| IBIS File main_fixed.ibs
| Cadence Design Systems, Inc. 2024
|[Doc Num]   FPGA-MD-02062 1.2
[IBIS ver]   3.2
[File name]   machxo3d.ibs
[File Rev]   0.8
[Date]   Mon Sep 23 20:28:33 PDT 2024
[Source]   Lattice Semiconductor cs200fl Process
[Notes]   Device: LCMXO3D-4300HC   Final
   Device: LCMXO3D-4300ZC   Final
   Device: LCMXO3D-9400HC   Final
   Device: LCMXO3D-9400ZC   Final
   Device: LCMXO3D-9400HE   Final
   Device: LAMXO3D-4300HC   Final
   Device: LAMXO3D-4300ZC   Final
   Device: LAMXO3D-9400HC   Final
   Device: LAMXO3D-9400ZC   Final
   Device: LAMXO3D-9400HE   Final
   "Test Release - internal Lattice use ONLY"
   Lattice Semiconductor has worked hard to ensure the
   models below are accurate and complete.  However, the
   data below was generated using simulation of the
   input/output model files for the silicon.  Therefore,
   the data below is for reference and initial design
   purposes only.
   Lattice Semiconductor grants permission to use this
   data for use in printed circuit design using this
   Lattice programmable logic device.  Other use of this
   code, including the selling or duplication of any
   portion is strictly prohibited.
|   NAMING CONVENTION
   The IBIS [Model] header is limited by the specification to a
   total of characters.  With such a set of characters available
   for naming models it becomes important to attempt to
   meaningfully encode the IO standards so they fit within the
   twenty character limit.  It would seem that twenty characters
   would provide room enough for describing IO's.  However, the
   PLD IO structure continues to grow more and more complex.  The
   complexity is making the twenty characters insuffiently
   descriptive.  In order to overcome this issue the naming
   convention described below is implemented to resolve the issue.
The twenty character space is managed as follows:
   bbbvvvsdddprugtcoixx
   b = standard
   v = voltage (x.xx V)
   s = slew code
   d = drive (xx.x ma)
   p = pullup code
   r = series resistance  or bank_vccio code
   u = terminate to vcc code
   g = terminate to gnd code
   t = terminate to vtt code
   c = common mode termination mode
   o = diff resistor code
   i = diff resistor current code
   x = reserved
   standard
   LVCMOS   lvc
   lvcmosd   lvd
   lvcmosr   lvr
   LVDS25E   lve
   LVTTL   lvt
   lvttld   ltd
   PCI   pci
   pcix   pcx
   lvds25   lvs
   blvds25   blv
   blvds25e   blv
   mlvds25   mlv
   mlvds25e   mle
   lvpecl   lvp
   lvpecl33   lvp
   lvpecl33e   lvp
   cml   cml
   hypt   hyp
   rsds25   rsd
   rsds25e   rse
   mipi_lp   mip
   mipi   mip
   vref1   vr1
   vref2   vr2
   ref_res   rer
   i3c33   i3c
   i3c18   i3c
   i3c12   i3c
   slew
   na   a
   fast   f
   slow   s
   pullmode
   off   a
   pullup   b
   pulldown   c
   bushold   d
   clamp   e
   up_clamp   f
   down_clamp   g
   keeper_clamp   h
   i3c_clamp   e
   impedance or Bank_vccio
   off   a
   25   b
   33   c
   50   d
   100   e
   3.3   f
   2.5   g
   1.8   h
   1.5   i
   1.2   j
   termVCC
   off   a
   50   b
   100   c
   120   d
   termGND
   off   a
   50   b
   100   c
   120   d
   termVTT
   off   a
   60   b
   75   c
   120   d
   150   e
   210   f
   VCMT
   off   a
   VCMT   b
   VTT   c
   DDR-2   d
   differential resistor
   off   a
   100   b
   diff drive
   NA   a
   2.0   b
   3.5   c
   1.25   f
   2.5   g
   Reserved   IO type
   in   input only
   ou   output
   io   I/O
   od   Open drain
   ic   Inverting differential input
   (signal name only)
   it   Non-Inverting differential
   input (signal name only)
   on   Inverting differential output
   (signal name only)
   op   Non-Inverting differential output
   (signal name only)
   bn   Inverting differential I/O
   (signal name only)
   bp   Non-Inverting differential I/O
   (signal name only)
   Lattice Semiconductor Corporation
   5555 NE Moore Court
   Hillsboro, OR 97214
   U.S.A
   TEL: 1-800-Lattice (USA and Canada)
   408-826-6000 (other locations)
   web: http://www.latticesemi.com/
   email: techsupport@latticesemi.com
[Disclaimer]  This IBIS source code is intended as a design reference which
  illustrates how the Lattice Semiconductor device operates. It is the user's
  responsibility to verify their design for consistency and functionality
  through the use of formal verification methods. Lattice Semiconductor
  provides no warranty regarding the use or functionality of this data.
[Copyright] Copyright 2024 by Lattice Semiconductor Corporation
|   Component XO3D
[Component] XO3D
[Manufacturer] Lattice Semiconductor Corp.
[Package]
|CABGA484
|variable   typ   min   max
R_pkg   262.26m   144.47m   388.32m
L_pkg   4.725nH   1.887nH   8.095nH
C_pkg   0.7093pF   0.3624pF   1.17pF
|CABGA400
|varibale   typ   min   max
|R_pkg   249.7m   145.37m   389.76m
|L_pkg   4.325nH   1.917nH   7.316nH
|C_pkg   0.6713pF   0.3727pF   1.207pF
|CABGA256_9400
|varibale   typ   min   max
|R_pkg   230.24m   185.88m   297.14m
|L_pkg   3.46nH   2.215nH   5.403nH
|C_pkg   0.5928pF   0.3835pF   0.8599pF
|QFN72_9400
|varibale   typ   min   max
|R_pkg   149.35m   99.917m   233.44m
|L_pkg   2.376nH   1.45nH   3.785nH
|C_pkg   0.3325pF   0.2601pF   0.4543pF
|CABGA256_4300
|variable   typ   min   max
|R_pkg   275.2m   212.49m   370.68m
|L_pkg   4.143nH   2.728nH   6.386nH
|C_pkg   0.654pF   0.4691pF   0.909pF
|QFN72_4300
|variable   typ   min   max
|R_pkg   175.42m   121.83m   245.44m
|L_pkg   2.78nH   1.676nH   3.852nH
|C_pkg   0.3626pF   0.28pF   0.4651pF
|WLCSP69_9400
|variable   typ   min   max
|R_pkg   241.03m   45.57m   642.53m
|L_pkg   0.721nH   0.213nH   1.601nH
|C_pkg   0.295pF   0.2333pF   0.4256pF
|FTBGA256
|variable   typ   min   max
|R_pkg   0.30461   0.20467   0.4353
|L_pkg   5.074e-9   2.654e-9   8.463e-9
|C_pkg   9.259e-13   7.079e-13   1.269e-12
[Pin]  signal_name   model_name   R_pin   L_pin   C_pin
1   blv250axxxafaaaaaait   blv250axxxafaaaaaain
2   blv250axxxafaaaaaaic   blv250axxxafaaaaaain
3   blv250axxxafaaaabait   blv250axxxafaaaabain
4   blv250axxxafaaaabaic   blv250axxxafaaaabain
5   blv250axxxagaaaaaait   blv250axxxagaaaaaain
6   blv250axxxagaaaaaaic   blv250axxxagaaaaaain
7   blv250axxxagaaaabait   blv250axxxagaaaabain
8   blv250axxxagaaaabaic   blv250axxxagaaaabain
9   blv250axxxefaaaaaait   blv250axxxefaaaaaain
10   blv250axxxefaaaaaaic   blv250axxxefaaaaaain
11   blv250axxxefaaaabait   blv250axxxefaaaabain
12   blv250axxxefaaaabaic   blv250axxxefaaaabain
13   blv250axxxegaaaaaait   blv250axxxegaaaaaain
14   blv250axxxegaaaaaaic   blv250axxxegaaaaaain
15   blv250axxxegaaaabait   blv250axxxegaaaabain
16   blv250axxxegaaaabaic   blv250axxxegaaaabain
17   blv250f160aaaaaaaabp   blv250f160aaaaaaaaio
18   blv250f160aaaaaaaabn   blv250f160aaaaaaaaio
19   blv250f160aaaaaaaaop   blv250f160aaaaaaaaou
20   blv250f160aaaaaaaaon   blv250f160aaaaaaaaou
21   blv250f160eaaaaaaabp   blv250f160eaaaaaaaio
22   blv250f160eaaaaaaabn   blv250f160eaaaaaaaio
23   blv250f160eaaaaaaaop   blv250f160eaaaaaaaou
24   blv250f160eaaaaaaaon   blv250f160eaaaaaaaou
25   blv250s160aaaaaaaabp   blv250s160aaaaaaaaio
26   blv250s160aaaaaaaabn   blv250s160aaaaaaaaio
27   blv250s160aaaaaaaaop   blv250s160aaaaaaaaou
28   blv250s160aaaaaaaaon   blv250s160aaaaaaaaou
29   blv250s160eaaaaaaabp   blv250s160eaaaaaaaio
30   blv250s160eaaaaaaabn   blv250s160eaaaaaaaio
31   blv250s160eaaaaaaaop   blv250s160eaaaaaaaou
32   blv250s160eaaaaaaaon   blv250s160eaaaaaaaou
33   i3c120f020aaaaaaaaio   i3c120f020aaaaaaaaio
34   i3c120f020eaaaaaaaio   i3c120f020eaaaaaaaio
35   i3c120s020aaaaaaaaio   i3c120s020aaaaaaaaio
36   i3c120s020eaaaaaaaio   i3c120s020eaaaaaaaio
37   i3c180f040aaaaaaaaio   i3c180f040aaaaaaaaio
38   i3c180f040eaaaaaaaio   i3c180f040eaaaaaaaio
39   i3c180s040aaaaaaaaio   i3c180s040aaaaaaaaio
40   i3c180s040eaaaaaaaio   i3c180s040eaaaaaaaio
41   i3c330f040aaaaaaaaio   i3c330f040aaaaaaaaio
42   i3c330f040eaaaaaaaio   i3c330f040eaaaaaaaio
43   i3c330s040aaaaaaaaio   i3c330s040aaaaaaaaio
44   i3c330s040eaaaaaaaio   i3c330s040eaaaaaaaio
45   ltd330axxxafaaaaaait   ltd330axxxafaaaaaain
46   ltd330axxxafaaaaaaic   ltd330axxxafaaaaaain
47   ltd330axxxefaaaaaait   ltd330axxxefaaaaaain
48   ltd330axxxefaaaaaaic   ltd330axxxefaaaaaain
49   ltd330f040aaaaaaaabp   ltd330f040aaaaaaaaio
50   ltd330f040aaaaaaaabn   ltd330f040aaaaaaaaio
51   ltd330f040aaaaaaaaop   ltd330f040aaaaaaaaou
52   ltd330f040aaaaaaaaon   ltd330f040aaaaaaaaou
53   ltd330f040eaaaaaaabp   ltd330f040eaaaaaaaio
54   ltd330f040eaaaaaaabn   ltd330f040eaaaaaaaio
55   ltd330f040eaaaaaaaop   ltd330f040eaaaaaaaou
56   ltd330f040eaaaaaaaon   ltd330f040eaaaaaaaou
57   ltd330f080aaaaaaaabp   ltd330f080aaaaaaaaio
58   ltd330f080aaaaaaaabn   ltd330f080aaaaaaaaio
59   ltd330f080aaaaaaaaop   ltd330f080aaaaaaaaou
60   ltd330f080aaaaaaaaon   ltd330f080aaaaaaaaou
61   ltd330f080eaaaaaaabp   ltd330f080eaaaaaaaio
62   ltd330f080eaaaaaaabn   ltd330f080eaaaaaaaio
63   ltd330f080eaaaaaaaop   ltd330f080eaaaaaaaou
64   ltd330f080eaaaaaaaon   ltd330f080eaaaaaaaou
65   ltd330f120aaaaaaaabp   ltd330f120aaaaaaaaio
66   ltd330f120aaaaaaaabn   ltd330f120aaaaaaaaio
67   ltd330f120aaaaaaaaop   ltd330f120aaaaaaaaou
68   ltd330f120aaaaaaaaon   ltd330f120aaaaaaaaou
69   ltd330f120eaaaaaaabp   ltd330f120eaaaaaaaio
70   ltd330f120eaaaaaaabn   ltd330f120eaaaaaaaio
71   ltd330f120eaaaaaaaop   ltd330f120eaaaaaaaou
72   ltd330f120eaaaaaaaon   ltd330f120eaaaaaaaou
73   ltd330f160aaaaaaaabp   ltd330f160aaaaaaaaio
74   ltd330f160aaaaaaaabn   ltd330f160aaaaaaaaio
75   ltd330f160aaaaaaaaop   ltd330f160aaaaaaaaou
76   ltd330f160aaaaaaaaon   ltd330f160aaaaaaaaou
77   ltd330f160eaaaaaaabp   ltd330f160eaaaaaaaio
78   ltd330f160eaaaaaaabn   ltd330f160eaaaaaaaio
79   ltd330f160eaaaaaaaop   ltd330f160eaaaaaaaou
80   ltd330f160eaaaaaaaon   ltd330f160eaaaaaaaou
81   ltd330s040aaaaaaaabp   ltd330s040aaaaaaaaio
82   ltd330s040aaaaaaaabn   ltd330s040aaaaaaaaio
83   ltd330s040aaaaaaaaop   ltd330s040aaaaaaaaou
84   ltd330s040aaaaaaaaon   ltd330s040aaaaaaaaou
85   ltd330s040eaaaaaaabp   ltd330s040eaaaaaaaio
86   ltd330s040eaaaaaaabn   ltd330s040eaaaaaaaio
87   ltd330s040eaaaaaaaop   ltd330s040eaaaaaaaou
88   ltd330s040eaaaaaaaon   ltd330s040eaaaaaaaou
89   ltd330s080aaaaaaaabp   ltd330s080aaaaaaaaio
90   ltd330s080aaaaaaaabn   ltd330s080aaaaaaaaio
91   ltd330s080aaaaaaaaop   ltd330s080aaaaaaaaou
92   ltd330s080aaaaaaaaon   ltd330s080aaaaaaaaou
93   ltd330s080eaaaaaaabp   ltd330s080eaaaaaaaio
94   ltd330s080eaaaaaaabn   ltd330s080eaaaaaaaio
95   ltd330s080eaaaaaaaop   ltd330s080eaaaaaaaou
96   ltd330s080eaaaaaaaon   ltd330s080eaaaaaaaou
97   ltd330s120aaaaaaaabp   ltd330s120aaaaaaaaio
98   ltd330s120aaaaaaaabn   ltd330s120aaaaaaaaio
99   ltd330s120aaaaaaaaop   ltd330s120aaaaaaaaou
100   ltd330s120aaaaaaaaon   ltd330s120aaaaaaaaou
101   ltd330s120eaaaaaaabp   ltd330s120eaaaaaaaio
102   ltd330s120eaaaaaaabn   ltd330s120eaaaaaaaio
103   ltd330s120eaaaaaaaop   ltd330s120eaaaaaaaou
104   ltd330s120eaaaaaaaon   ltd330s120eaaaaaaaou
105   ltd330s160aaaaaaaabp   ltd330s160aaaaaaaaio
106   ltd330s160aaaaaaaabn   ltd330s160aaaaaaaaio
107   ltd330s160aaaaaaaaop   ltd330s160aaaaaaaaou
108   ltd330s160aaaaaaaaon   ltd330s160aaaaaaaaou
109   ltd330s160eaaaaaaabp   ltd330s160eaaaaaaaio
110   ltd330s160eaaaaaaabn   ltd330s160eaaaaaaaio
111   ltd330s160eaaaaaaaop   ltd330s160eaaaaaaaou
112   ltd330s160eaaaaaaaon   ltd330s160eaaaaaaaou
113   lvc120axxxafaaaaaain   lvc120axxxafaaaaaain
114   lvc120axxxagaaaaaain   lvc120axxxagaaaaaain
115   lvc120axxxahaaaaaain   lvc120axxxahaaaaaain
116   lvc120axxxaiaaaaaain   lvc120axxxaiaaaaaain
117   lvc120axxxbjaaaaaain   lvc120axxxbjaaaaaain
118   lvc120axxxcfaaaaaain   lvc120axxxcfaaaaaain
119   lvc120axxxcgaaaaaain   lvc120axxxcgaaaaaain
120   lvc120axxxchaaaaaain   lvc120axxxchaaaaaain
121   lvc120axxxciaaaaaain   lvc120axxxciaaaaaain
122   lvc120axxxdjaaaaaain   lvc120axxxdjaaaaaain
123   lvc120axxxefaaaaaain   lvc120axxxefaaaaaain
124   lvc120axxxegaaaaaain   lvc120axxxegaaaaaain
125   lvc120axxxehaaaaaain   lvc120axxxehaaaaaain
126   lvc120axxxeiaaaaaain   lvc120axxxeiaaaaaain
127   lvc120axxxejaaaaaain   lvc120axxxejaaaaaain
128   lvc120axxxfjaaaaaain   lvc120axxxfjaaaaaain
129   lvc120axxxgfaaaaaain   lvc120axxxgfaaaaaain
130   lvc120axxxggaaaaaain   lvc120axxxggaaaaaain
131   lvc120axxxghaaaaaain   lvc120axxxghaaaaaain
132   lvc120axxxgiaaaaaain   lvc120axxxgiaaaaaain
133   lvc120axxxgjaaaaaain   lvc120axxxgjaaaaaain
134   lvc120axxxhjaaaaaain   lvc120axxxhjaaaaaain
135   lvc120f020aaaaaaaaio   lvc120f020aaaaaaaaio
136   lvc120f020aaaaaaaaou   lvc120f020aaaaaaaaou
137   lvc120f020baaaaaaaio   lvc120f020baaaaaaaio
138   lvc120f020baaaaaaaou   lvc120f020baaaaaaaou
139   lvc120f020caaaaaaaio   lvc120f020caaaaaaaio
140   lvc120f020caaaaaaaou   lvc120f020caaaaaaaou
141   lvc120f020daaaaaaaio   lvc120f020daaaaaaaio
142   lvc120f020daaaaaaaou   lvc120f020daaaaaaaou
143   lvc120f020eaaaaaaaio   lvc120f020eaaaaaaaio
144   lvc120f020eaaaaaaaou   lvc120f020eaaaaaaaou
145   lvc120f020faaaaaaaio   lvc120f020faaaaaaaio
146   lvc120f020faaaaaaaou   lvc120f020faaaaaaaou
147   lvc120f020gaaaaaaaio   lvc120f020gaaaaaaaio
148   lvc120f020gaaaaaaaou   lvc120f020gaaaaaaaou
149   lvc120f020haaaaaaaio   lvc120f020haaaaaaaio
150   lvc120f020haaaaaaaou   lvc120f020haaaaaaaou
151   lvc120f040afaaaaaaod   lvc120f040afaaaaaaod
152   lvc120f040agaaaaaaod   lvc120f040agaaaaaaod
153   lvc120f040ahaaaaaaod   lvc120f040ahaaaaaaod
154   lvc120f040aiaaaaaaod   lvc120f040aiaaaaaaod
155   lvc120f040ajaaaaaaod   lvc120f040ajaaaaaaod
156   lvc120f060aaaaaaaaio   lvc120f060aaaaaaaaio
157   lvc120f060aaaaaaaaou   lvc120f060aaaaaaaaou
158   lvc120f060baaaaaaaio   lvc120f060baaaaaaaio
159   lvc120f060baaaaaaaou   lvc120f060baaaaaaaou
160   lvc120f060caaaaaaaio   lvc120f060caaaaaaaio
161   lvc120f060caaaaaaaou   lvc120f060caaaaaaaou
162   lvc120f060daaaaaaaio   lvc120f060daaaaaaaio
163   lvc120f060daaaaaaaou   lvc120f060daaaaaaaou
164   lvc120f060eaaaaaaaio   lvc120f060eaaaaaaaio
165   lvc120f060eaaaaaaaou   lvc120f060eaaaaaaaou
166   lvc120f060faaaaaaaio   lvc120f060faaaaaaaio
167   lvc120f060faaaaaaaou   lvc120f060faaaaaaaou
168   lvc120f060gaaaaaaaio   lvc120f060gaaaaaaaio
169   lvc120f060gaaaaaaaou   lvc120f060gaaaaaaaou
170   lvc120f060haaaaaaaio   lvc120f060haaaaaaaio
171   lvc120f060haaaaaaaou   lvc120f060haaaaaaaou
172   lvc120f080afaaaaaaod   lvc120f080afaaaaaaod
173   lvc120f080agaaaaaaod   lvc120f080agaaaaaaod
174   lvc120f080ahaaaaaaod   lvc120f080ahaaaaaaod
175   lvc120f080aiaaaaaaod   lvc120f080aiaaaaaaod
176   lvc120f080ajaaaaaaod   lvc120f080ajaaaaaaod
177   lvc120f120afaaaaaaod   lvc120f120afaaaaaaod
178   lvc120f120agaaaaaaod   lvc120f120agaaaaaaod
179   lvc120f120ahaaaaaaod   lvc120f120ahaaaaaaod
180   lvc120f160afaaaaaaod   lvc120f160afaaaaaaod
181   lvc120f160agaaaaaaod   lvc120f160agaaaaaaod
182   lvc120s020aaaaaaaaio   lvc120s020aaaaaaaaio
183   lvc120s020aaaaaaaaou   lvc120s020aaaaaaaaou
184   lvc120s020baaaaaaaio   lvc120s020baaaaaaaio
185   lvc120s020baaaaaaaou   lvc120s020baaaaaaaou
186   lvc120s020caaaaaaaio   lvc120s020caaaaaaaio
187   lvc120s020caaaaaaaou   lvc120s020caaaaaaaou
188   lvc120s020daaaaaaaio   lvc120s020daaaaaaaio
189   lvc120s020daaaaaaaou   lvc120s020daaaaaaaou
190   lvc120s020eaaaaaaaio   lvc120s020eaaaaaaaio
191   lvc120s020eaaaaaaaou   lvc120s020eaaaaaaaou
192   lvc120s020faaaaaaaio   lvc120s020faaaaaaaio
193   lvc120s020faaaaaaaou   lvc120s020faaaaaaaou
194   lvc120s020gaaaaaaaio   lvc120s020gaaaaaaaio
195   lvc120s020gaaaaaaaou   lvc120s020gaaaaaaaou
196   lvc120s020haaaaaaaio   lvc120s020haaaaaaaio
197   lvc120s020haaaaaaaou   lvc120s020haaaaaaaou
198   lvc120s040afaaaaaaod   lvc120s040afaaaaaaod
199   lvc120s040agaaaaaaod   lvc120s040agaaaaaaod
200   lvc120s040ahaaaaaaod   lvc120s040ahaaaaaaod
201   lvc120s040aiaaaaaaod   lvc120s040aiaaaaaaod
202   lvc120s040ajaaaaaaod   lvc120s040ajaaaaaaod
203   lvc120s060aaaaaaaaio   lvc120s060aaaaaaaaio
204   lvc120s060aaaaaaaaou   lvc120s060aaaaaaaaou
205   lvc120s060baaaaaaaio   lvc120s060baaaaaaaio
206   lvc120s060baaaaaaaou   lvc120s060baaaaaaaou
207   lvc120s060caaaaaaaio   lvc120s060caaaaaaaio
208   lvc120s060caaaaaaaou   lvc120s060caaaaaaaou
209   lvc120s060daaaaaaaio   lvc120s060daaaaaaaio
210   lvc120s060daaaaaaaou   lvc120s060daaaaaaaou
211   lvc120s060eaaaaaaaio   lvc120s060eaaaaaaaio
212   lvc120s060eaaaaaaaou   lvc120s060eaaaaaaaou
213   lvc120s060faaaaaaaio   lvc120s060faaaaaaaio
214   lvc120s060faaaaaaaou   lvc120s060faaaaaaaou
215   lvc120s060gaaaaaaaio   lvc120s060gaaaaaaaio
216   lvc120s060gaaaaaaaou   lvc120s060gaaaaaaaou
217   lvc120s060haaaaaaaio   lvc120s060haaaaaaaio
218   lvc120s060haaaaaaaou   lvc120s060haaaaaaaou
219   lvc120s080afaaaaaaod   lvc120s080afaaaaaaod
220   lvc120s080agaaaaaaod   lvc120s080agaaaaaaod
221   lvc120s080ahaaaaaaod   lvc120s080ahaaaaaaod
222   lvc120s080aiaaaaaaod   lvc120s080aiaaaaaaod
223   lvc120s080ajaaaaaaod   lvc120s080ajaaaaaaod
224   lvc120s120afaaaaaaod   lvc120s120afaaaaaaod
225   lvc120s120agaaaaaaod   lvc120s120agaaaaaaod
226   lvc120s120ahaaaaaaod   lvc120s120ahaaaaaaod
227   lvc120s160afaaaaaaod   lvc120s160afaaaaaaod
228   lvc120s160agaaaaaaod   lvc120s160agaaaaaaod
229   lvc150axxxafaaaaaain   lvc150axxxafaaaaaain
230   lvc150axxxagaaaaaain   lvc150axxxagaaaaaain
231   lvc150axxxahaaaaaain   lvc150axxxahaaaaaain
232   lvc150axxxaiaaaaaain   lvc150axxxaiaaaaaain
233   lvc150axxxajaaaaaain   lvc150axxxajaaaaaain
234   lvc150axxxbiaaaaaain   lvc150axxxbiaaaaaain
235   lvc150axxxcfaaaaaain   lvc150axxxcfaaaaaain
236   lvc150axxxcgaaaaaain   lvc150axxxcgaaaaaain
237   lvc150axxxchaaaaaain   lvc150axxxchaaaaaain
238   lvc150axxxciaaaaaain   lvc150axxxciaaaaaain
239   lvc150axxxcjaaaaaain   lvc150axxxcjaaaaaain
240   lvc150axxxdiaaaaaain   lvc150axxxdiaaaaaain
241   lvc150axxxefaaaaaain   lvc150axxxefaaaaaain
242   lvc150axxxegaaaaaain   lvc150axxxegaaaaaain
243   lvc150axxxehaaaaaain   lvc150axxxehaaaaaain
244   lvc150axxxeiaaaaaain   lvc150axxxeiaaaaaain
245   lvc150axxxfiaaaaaain   lvc150axxxfiaaaaaain
246   lvc150axxxgfaaaaaain   lvc150axxxgfaaaaaain
247   lvc150axxxggaaaaaain   lvc150axxxggaaaaaain
248   lvc150axxxghaaaaaain   lvc150axxxghaaaaaain
249   lvc150axxxgiaaaaaain   lvc150axxxgiaaaaaain
250   lvc150axxxhiaaaaaain   lvc150axxxhiaaaaaain
251   lvc150f040afaaaaaaod   lvc150f040afaaaaaaod
252   lvc150f040agaaaaaaod   lvc150f040agaaaaaaod
253   lvc150f040ahaaaaaaod   lvc150f040ahaaaaaaod
254   lvc150f040aaaaaaaaio   lvc150f040aaaaaaaaio
255   lvc150f040aiaaaaaaod   lvc150f040aiaaaaaaod
256   lvc150f040aaaaaaaaou   lvc150f040aaaaaaaaou
257   lvc150f040ajaaaaaaod   lvc150f040ajaaaaaaod
258   lvc150f040baaaaaaaio   lvc150f040baaaaaaaio
259   lvc150f040baaaaaaaou   lvc150f040baaaaaaaou
260   lvc150f040caaaaaaaio   lvc150f040caaaaaaaio
261   lvc150f040caaaaaaaou   lvc150f040caaaaaaaou
262   lvc150f040daaaaaaaio   lvc150f040daaaaaaaio
263   lvc150f040daaaaaaaou   lvc150f040daaaaaaaou
264   lvc150f040eaaaaaaaio   lvc150f040eaaaaaaaio
265   lvc150f040eaaaaaaaou   lvc150f040eaaaaaaaou
266   lvc150f040faaaaaaaio   lvc150f040faaaaaaaio
267   lvc150f040faaaaaaaou   lvc150f040faaaaaaaou
268   lvc150f040gaaaaaaaio   lvc150f040gaaaaaaaio
269   lvc150f040gaaaaaaaou   lvc150f040gaaaaaaaou
270   lvc150f040haaaaaaaio   lvc150f040haaaaaaaio
271   lvc150f040haaaaaaaou   lvc150f040haaaaaaaou
272   lvc150f080afaaaaaaod   lvc150f080afaaaaaaod
273   lvc150f080agaaaaaaod   lvc150f080agaaaaaaod
274   lvc150f080ahaaaaaaod   lvc150f080ahaaaaaaod
275   lvc150f080aaaaaaaaio   lvc150f080aaaaaaaaio
276   lvc150f080aiaaaaaaod   lvc150f080aiaaaaaaod
277   lvc150f080aaaaaaaaou   lvc150f080aaaaaaaaou
278   lvc150f080ajaaaaaaod   lvc150f080ajaaaaaaod
279   lvc150f080baaaaaaaio   lvc150f080baaaaaaaio
280   lvc150f080baaaaaaaou   lvc150f080baaaaaaaou
281   lvc150f080caaaaaaaio   lvc150f080caaaaaaaio
282   lvc150f080caaaaaaaou   lvc150f080caaaaaaaou
283   lvc150f080daaaaaaaio   lvc150f080daaaaaaaio
284   lvc150f080daaaaaaaou   lvc150f080daaaaaaaou
285   lvc150f080eaaaaaaaio   lvc150f080eaaaaaaaio
286   lvc150f080eaaaaaaaou   lvc150f080eaaaaaaaou
287   lvc150f080faaaaaaaio   lvc150f080faaaaaaaio
288   lvc150f080faaaaaaaou   lvc150f080faaaaaaaou
289   lvc150f080gaaaaaaaio   lvc150f080gaaaaaaaio
290   lvc150f080gaaaaaaaou   lvc150f080gaaaaaaaou
291   lvc150f080haaaaaaaio   lvc150f080haaaaaaaio
292   lvc150f080haaaaaaaou   lvc150f080haaaaaaaou
293   lvc150f120afaaaaaaod   lvc150f120afaaaaaaod
294   lvc150f120agaaaaaaod   lvc150f120agaaaaaaod
295   lvc150f120ahaaaaaaod   lvc150f120ahaaaaaaod
296   lvc150f160afaaaaaaod   lvc150f160afaaaaaaod
297   lvc150f160agaaaaaaod   lvc150f160agaaaaaaod
298   lvc150s040afaaaaaaod   lvc150s040afaaaaaaod
299   lvc150s040agaaaaaaod   lvc150s040agaaaaaaod
300   lvc150s040ahaaaaaaod   lvc150s040ahaaaaaaod
301   lvc150s040aaaaaaaaio   lvc150s040aaaaaaaaio
302   lvc150s040aiaaaaaaod   lvc150s040aiaaaaaaod
303   lvc150s040aaaaaaaaou   lvc150s040aaaaaaaaou
304   lvc150s040ajaaaaaaod   lvc150s040ajaaaaaaod
305   lvc150s040baaaaaaaio   lvc150s040baaaaaaaio
306   lvc150s040baaaaaaaou   lvc150s040baaaaaaaou
307   lvc150s040caaaaaaaio   lvc150s040caaaaaaaio
308   lvc150s040caaaaaaaou   lvc150s040caaaaaaaou
309   lvc150s040daaaaaaaio   lvc150s040daaaaaaaio
310   lvc150s040daaaaaaaou   lvc150s040daaaaaaaou
311   lvc150s040eaaaaaaaio   lvc150s040eaaaaaaaio
312   lvc150s040eaaaaaaaou   lvc150s040eaaaaaaaou
313   lvc150s040faaaaaaaio   lvc150s040faaaaaaaio
314   lvc150s040faaaaaaaou   lvc150s040faaaaaaaou
315   lvc150s040gaaaaaaaio   lvc150s040gaaaaaaaio
316   lvc150s040gaaaaaaaou   lvc150s040gaaaaaaaou
317   lvc150s040haaaaaaaio   lvc150s040haaaaaaaio
318   lvc150s040haaaaaaaou   lvc150s040haaaaaaaou
319   lvc150s080afaaaaaaod   lvc150s080afaaaaaaod
320   lvc150s080agaaaaaaod   lvc150s080agaaaaaaod
321   lvc150s080ahaaaaaaod   lvc150s080ahaaaaaaod
322   lvc150s080aaaaaaaaio   lvc150s080aaaaaaaaio
323   lvc150s080aiaaaaaaod   lvc150s080aiaaaaaaod
324   lvc150s080aaaaaaaaou   lvc150s080aaaaaaaaou
325   lvc150s080ajaaaaaaod   lvc150s080ajaaaaaaod
326   lvc150s080baaaaaaaio   lvc150s080baaaaaaaio
327   lvc150s080baaaaaaaou   lvc150s080baaaaaaaou
328   lvc150s080caaaaaaaio   lvc150s080caaaaaaaio
329   lvc150s080caaaaaaaou   lvc150s080caaaaaaaou
330   lvc150s080daaaaaaaio   lvc150s080daaaaaaaio
331   lvc150s080daaaaaaaou   lvc150s080daaaaaaaou
332   lvc150s080eaaaaaaaio   lvc150s080eaaaaaaaio
333   lvc150s080eaaaaaaaou   lvc150s080eaaaaaaaou
334   lvc150s080faaaaaaaio   lvc150s080faaaaaaaio
335   lvc150s080faaaaaaaou   lvc150s080faaaaaaaou
336   lvc150s080gaaaaaaaio   lvc150s080gaaaaaaaio
337   lvc150s080gaaaaaaaou   lvc150s080gaaaaaaaou
338   lvc150s080haaaaaaaio   lvc150s080haaaaaaaio
339   lvc150s080haaaaaaaou   lvc150s080haaaaaaaou
340   lvc150s120afaaaaaaod   lvc150s120afaaaaaaod
341   lvc150s120agaaaaaaod   lvc150s120agaaaaaaod
342   lvc150s120ahaaaaaaod   lvc150s120ahaaaaaaod
343   lvc150s160afaaaaaaod   lvc150s160afaaaaaaod
344   lvc150s160agaaaaaaod   lvc150s160agaaaaaaod
345   lvc180axxxafaaaaaain   lvc180axxxafaaaaaain
346   lvc180axxxagaaaaaain   lvc180axxxagaaaaaain
347   lvc180axxxahaaaaaain   lvc180axxxahaaaaaain
348   lvc180axxxaiaaaaaain   lvc180axxxaiaaaaaain
349   lvc180axxxbhaaaaaain   lvc180axxxbhaaaaaain
350   lvc180axxxcfaaaaaain   lvc180axxxcfaaaaaain
351   lvc180axxxcgaaaaaain   lvc180axxxcgaaaaaain
352   lvc180axxxchaaaaaain   lvc180axxxchaaaaaain
353   lvc180axxxciaaaaaain   lvc180axxxciaaaaaain
354   lvc180axxxdhaaaaaain   lvc180axxxdhaaaaaain
355   lvc180axxxefaaaaaain   lvc180axxxefaaaaaain
356   lvc180axxxegaaaaaain   lvc180axxxegaaaaaain
357   lvc180axxxehaaaaaain   lvc180axxxehaaaaaain
358   lvc180axxxfhaaaaaain   lvc180axxxfhaaaaaain
359   lvc180axxxgfaaaaaain   lvc180axxxgfaaaaaain
360   lvc180axxxggaaaaaain   lvc180axxxggaaaaaain
361   lvc180axxxghaaaaaain   lvc180axxxghaaaaaain
362   lvc180axxxhhaaaaaain   lvc180axxxhhaaaaaain
363   lvc180f040afaaaaaaod   lvc180f040afaaaaaaod
364   lvc180f040agaaaaaaod   lvc180f040agaaaaaaod
365   lvc180f040aaaaaaaaio   lvc180f040aaaaaaaaio
366   lvc180f040ahaaaaaaod   lvc180f040ahaaaaaaod
367   lvc180f040aaaaaaaaou   lvc180f040aaaaaaaaou
368   lvc180f040aiaaaaaaod   lvc180f040aiaaaaaaod
369   lvc180f040ajaaaaaaod   lvc180f040ajaaaaaaod
370   lvc180f040baaaaaaaio   lvc180f040baaaaaaaio
371   lvc180f040baaaaaaaou   lvc180f040baaaaaaaou
372   lvc180f040caaaaaaaio   lvc180f040caaaaaaaio
373   lvc180f040caaaaaaaou   lvc180f040caaaaaaaou
374   lvc180f040daaaaaaaio   lvc180f040daaaaaaaio
375   lvc180f040daaaaaaaou   lvc180f040daaaaaaaou
376   lvc180f040eaaaaaaaio   lvc180f040eaaaaaaaio
377   lvc180f040eaaaaaaaou   lvc180f040eaaaaaaaou
378   lvc180f040faaaaaaaio   lvc180f040faaaaaaaio
379   lvc180f040faaaaaaaou   lvc180f040faaaaaaaou
380   lvc180f040gaaaaaaaio   lvc180f040gaaaaaaaio
381   lvc180f040gaaaaaaaou   lvc180f040gaaaaaaaou
382   lvc180f040haaaaaaaio   lvc180f040haaaaaaaio
383   lvc180f040haaaaaaaou   lvc180f040haaaaaaaou
384   lvc180f080afaaaaaaod   lvc180f080afaaaaaaod
385   lvc180f080agaaaaaaod   lvc180f080agaaaaaaod
386   lvc180f080aaaaaaaaio   lvc180f080aaaaaaaaio
387   lvc180f080ahaaaaaaod   lvc180f080ahaaaaaaod
388   lvc180f080aaaaaaaaou   lvc180f080aaaaaaaaou
389   lvc180f080aiaaaaaaod   lvc180f080aiaaaaaaod
390   lvc180f080ajaaaaaaod   lvc180f080ajaaaaaaod
391   lvc180f080baaaaaaaio   lvc180f080baaaaaaaio
392   lvc180f080baaaaaaaou   lvc180f080baaaaaaaou
393   lvc180f080caaaaaaaio   lvc180f080caaaaaaaio
394   lvc180f080caaaaaaaou   lvc180f080caaaaaaaou
395   lvc180f080daaaaaaaio   lvc180f080daaaaaaaio
396   lvc180f080daaaaaaaou   lvc180f080daaaaaaaou
397   lvc180f080eaaaaaaaio   lvc180f080eaaaaaaaio
398   lvc180f080eaaaaaaaou   lvc180f080eaaaaaaaou
399   lvc180f080faaaaaaaio   lvc180f080faaaaaaaio
400   lvc180f080faaaaaaaou   lvc180f080faaaaaaaou
401   lvc180f080gaaaaaaaio   lvc180f080gaaaaaaaio
402   lvc180f080gaaaaaaaou   lvc180f080gaaaaaaaou
403   lvc180f080haaaaaaaio   lvc180f080haaaaaaaio
404   lvc180f080haaaaaaaou   lvc180f080haaaaaaaou
405   lvc180f120afaaaaaaod   lvc180f120afaaaaaaod
406   lvc180f120agaaaaaaod   lvc180f120agaaaaaaod
407   lvc180f120aaaaaaaaio   lvc180f120aaaaaaaaio
408   lvc180f120ahaaaaaaod   lvc180f120ahaaaaaaod
409   lvc180f120aaaaaaaaou   lvc180f120aaaaaaaaou
410   lvc180f120baaaaaaaio   lvc180f120baaaaaaaio
411   lvc180f120baaaaaaaou   lvc180f120baaaaaaaou
412   lvc180f120caaaaaaaio   lvc180f120caaaaaaaio
413   lvc180f120caaaaaaaou   lvc180f120caaaaaaaou
414   lvc180f120daaaaaaaio   lvc180f120daaaaaaaio
415   lvc180f120daaaaaaaou   lvc180f120daaaaaaaou
416   lvc180f120eaaaaaaaio   lvc180f120eaaaaaaaio
417   lvc180f120eaaaaaaaou   lvc180f120eaaaaaaaou
418   lvc180f120faaaaaaaio   lvc180f120faaaaaaaio
419   lvc180f120faaaaaaaou   lvc180f120faaaaaaaou
420   lvc180f120gaaaaaaaio   lvc180f120gaaaaaaaio
421   lvc180f120gaaaaaaaou   lvc180f120gaaaaaaaou
422   lvc180f120haaaaaaaio   lvc180f120haaaaaaaio
423   lvc180f120haaaaaaaou   lvc180f120haaaaaaaou
424   lvc180f160afaaaaaaod   lvc180f160afaaaaaaod
425   lvc180f160agaaaaaaod   lvc180f160agaaaaaaod
426   lvc180s040afaaaaaaod   lvc180s040afaaaaaaod
427   lvc180s040agaaaaaaod   lvc180s040agaaaaaaod
428   lvc180s040aaaaaaaaio   lvc180s040aaaaaaaaio
429   lvc180s040ahaaaaaaod   lvc180s040ahaaaaaaod
430   lvc180s040aaaaaaaaou   lvc180s040aaaaaaaaou
431   lvc180s040aiaaaaaaod   lvc180s040aiaaaaaaod
432   lvc180s040ajaaaaaaod   lvc180s040ajaaaaaaod
433   lvc180s040baaaaaaaio   lvc180s040baaaaaaaio
434   lvc180s040baaaaaaaou   lvc180s040baaaaaaaou
435   lvc180s040caaaaaaaio   lvc180s040caaaaaaaio
436   lvc180s040caaaaaaaou   lvc180s040caaaaaaaou
437   lvc180s040daaaaaaaio   lvc180s040daaaaaaaio
438   lvc180s040daaaaaaaou   lvc180s040daaaaaaaou
439   lvc180s040eaaaaaaaio   lvc180s040eaaaaaaaio
440   lvc180s040eaaaaaaaou   lvc180s040eaaaaaaaou
441   lvc180s040faaaaaaaio   lvc180s040faaaaaaaio
442   lvc180s040faaaaaaaou   lvc180s040faaaaaaaou
443   lvc180s040gaaaaaaaio   lvc180s040gaaaaaaaio
444   lvc180s040gaaaaaaaou   lvc180s040gaaaaaaaou
445   lvc180s040haaaaaaaio   lvc180s040haaaaaaaio
446   lvc180s040haaaaaaaou   lvc180s040haaaaaaaou
447   lvc180s080afaaaaaaod   lvc180s080afaaaaaaod
448   lvc180s080agaaaaaaod   lvc180s080agaaaaaaod
449   lvc180s080aaaaaaaaio   lvc180s080aaaaaaaaio
450   lvc180s080ahaaaaaaod   lvc180s080ahaaaaaaod
451   lvc180s080aaaaaaaaou   lvc180s080aaaaaaaaou
452   lvc180s080aiaaaaaaod   lvc180s080aiaaaaaaod
453   lvc180s080ajaaaaaaod   lvc180s080ajaaaaaaod
454   lvc180s080baaaaaaaio   lvc180s080baaaaaaaio
455   lvc180s080baaaaaaaou   lvc180s080baaaaaaaou
456   lvc180s080caaaaaaaio   lvc180s080caaaaaaaio
457   lvc180s080caaaaaaaou   lvc180s080caaaaaaaou
458   lvc180s080daaaaaaaio   lvc180s080daaaaaaaio
459   lvc180s080daaaaaaaou   lvc180s080daaaaaaaou
460   lvc180s080eaaaaaaaio   lvc180s080eaaaaaaaio
461   lvc180s080eaaaaaaaou   lvc180s080eaaaaaaaou
462   lvc180s080faaaaaaaio   lvc180s080faaaaaaaio
463   lvc180s080faaaaaaaou   lvc180s080faaaaaaaou
464   lvc180s080gaaaaaaaio   lvc180s080gaaaaaaaio
465   lvc180s080gaaaaaaaou   lvc180s080gaaaaaaaou
466   lvc180s080haaaaaaaio   lvc180s080haaaaaaaio
467   lvc180s080haaaaaaaou   lvc180s080haaaaaaaou
468   lvc180s120afaaaaaaod   lvc180s120afaaaaaaod
469   lvc180s120agaaaaaaod   lvc180s120agaaaaaaod
470   lvc180s120aaaaaaaaio   lvc180s120aaaaaaaaio
471   lvc180s120ahaaaaaaod   lvc180s120ahaaaaaaod
472   lvc180s120aaaaaaaaou   lvc180s120aaaaaaaaou
473   lvc180s120baaaaaaaio   lvc180s120baaaaaaaio
474   lvc180s120baaaaaaaou   lvc180s120baaaaaaaou
475   lvc180s120caaaaaaaio   lvc180s120caaaaaaaio
476   lvc180s120caaaaaaaou   lvc180s120caaaaaaaou
477   lvc180s120daaaaaaaio   lvc180s120daaaaaaaio
478   lvc180s120daaaaaaaou   lvc180s120daaaaaaaou
479   lvc180s120eaaaaaaaio   lvc180s120eaaaaaaaio
480   lvc180s120eaaaaaaaou   lvc180s120eaaaaaaaou
481   lvc180s120faaaaaaaio   lvc180s120faaaaaaaio
482   lvc180s120faaaaaaaou   lvc180s120faaaaaaaou
483   lvc180s120gaaaaaaaio   lvc180s120gaaaaaaaio
484   lvc180s120gaaaaaaaou   lvc180s120gaaaaaaaou
485   lvc180s120haaaaaaaio   lvc180s120haaaaaaaio
486   lvc180s120haaaaaaaou   lvc180s120haaaaaaaou
487   lvc180s160afaaaaaaod   lvc180s160afaaaaaaod
488   lvc180s160agaaaaaaod   lvc180s160agaaaaaaod
489   lvc250axxxafaaaaaain   lvc250axxxafaaaaaain
490   lvc250axxxagaaaaaain   lvc250axxxagaaaaaain
491   lvc250axxxahaaaaaain   lvc250axxxahaaaaaain
492   lvc250axxxaiaaaaaain   lvc250axxxaiaaaaaain
493   lvc250axxxbgaaaaaain   lvc250axxxbgaaaaaain
494   lvc250axxxcfaaaaaain   lvc250axxxcfaaaaaain
495   lvc250axxxcgaaaaaain   lvc250axxxcgaaaaaain
496   lvc250axxxchaaaaaain   lvc250axxxchaaaaaain
497   lvc250axxxciaaaaaain   lvc250axxxciaaaaaain
498   lvc250axxxdgaaaaaain   lvc250axxxdgaaaaaain
499   lvc250axxxegaaaaaain   lvc250axxxegaaaaaain
500   lvc250axxxfgaaaaaain   lvc250axxxfgaaaaaain
501   lvc250axxxggaaaaaain   lvc250axxxggaaaaaain
502   lvc250axxxhgaaaaaain   lvc250axxxhgaaaaaain
503   lvc250f040afaaaaaaod   lvc250f040afaaaaaaod
504   lvc250f040aaaaaaaaio   lvc250f040aaaaaaaaio
505   lvc250f040agaaaaaaod   lvc250f040agaaaaaaod
506   lvc250f040aaaaaaaaou   lvc250f040aaaaaaaaou
507   lvc250f040ahaaaaaaod   lvc250f040ahaaaaaaod
508   lvc250f040aiaaaaaaod   lvc250f040aiaaaaaaod
509   lvc250f040ajaaaaaaod   lvc250f040ajaaaaaaod
510   lvc250f040baaaaaaaio   lvc250f040baaaaaaaio
511   lvc250f040baaaaaaaou   lvc250f040baaaaaaaou
512   lvc250f040caaaaaaaio   lvc250f040caaaaaaaio
513   lvc250f040caaaaaaaou   lvc250f040caaaaaaaou
514   lvc250f040daaaaaaaio   lvc250f040daaaaaaaio
515   lvc250f040daaaaaaaou   lvc250f040daaaaaaaou
516   lvc250f040eaaaaaaaio   lvc250f040eaaaaaaaio
517   lvc250f040eaaaaaaaou   lvc250f040eaaaaaaaou
518   lvc250f040faaaaaaaio   lvc250f040faaaaaaaio
519   lvc250f040faaaaaaaou   lvc250f040faaaaaaaou
520   lvc250f040gaaaaaaaio   lvc250f040gaaaaaaaio
521   lvc250f040gaaaaaaaou   lvc250f040gaaaaaaaou
522   lvc250f040haaaaaaaio   lvc250f040haaaaaaaio
523   lvc250f040haaaaaaaou   lvc250f040haaaaaaaou
524   lvc250f080afaaaaaaod   lvc250f080afaaaaaaod
525   lvc250f080aaaaaaaaio   lvc250f080aaaaaaaaio
526   lvc250f080agaaaaaaod   lvc250f080agaaaaaaod
527   lvc250f080aaaaaaaaou   lvc250f080aaaaaaaaou
528   lvc250f080ahaaaaaaod   lvc250f080ahaaaaaaod
529   lvc250f080aiaaaaaaod   lvc250f080aiaaaaaaod
530   lvc250f080ajaaaaaaod   lvc250f080ajaaaaaaod
531   lvc250f080baaaaaaaio   lvc250f080baaaaaaaio
532   lvc250f080baaaaaaaou   lvc250f080baaaaaaaou
533   lvc250f080caaaaaaaio   lvc250f080caaaaaaaio
534   lvc250f080caaaaaaaou   lvc250f080caaaaaaaou
535   lvc250f080daaaaaaaio   lvc250f080daaaaaaaio
536   lvc250f080daaaaaaaou   lvc250f080daaaaaaaou
537   lvc250f080eaaaaaaaio   lvc250f080eaaaaaaaio
538   lvc250f080eaaaaaaaou   lvc250f080eaaaaaaaou
539   lvc250f080faaaaaaaio   lvc250f080faaaaaaaio
540   lvc250f080faaaaaaaou   lvc250f080faaaaaaaou
541   lvc250f080gaaaaaaaio   lvc250f080gaaaaaaaio
542   lvc250f080gaaaaaaaou   lvc250f080gaaaaaaaou
543   lvc250f080haaaaaaaio   lvc250f080haaaaaaaio
544   lvc250f080haaaaaaaou   lvc250f080haaaaaaaou
545   lvc250f120afaaaaaaod   lvc250f120afaaaaaaod
546   lvc250f120aaaaaaaaio   lvc250f120aaaaaaaaio
547   lvc250f120agaaaaaaod   lvc250f120agaaaaaaod
548   lvc250f120aaaaaaaaou   lvc250f120aaaaaaaaou
549   lvc250f120ahaaaaaaod   lvc250f120ahaaaaaaod
550   lvc250f120baaaaaaaio   lvc250f120baaaaaaaio
551   lvc250f120baaaaaaaou   lvc250f120baaaaaaaou
552   lvc250f120caaaaaaaio   lvc250f120caaaaaaaio
553   lvc250f120caaaaaaaou   lvc250f120caaaaaaaou
554   lvc250f120daaaaaaaio   lvc250f120daaaaaaaio
555   lvc250f120daaaaaaaou   lvc250f120daaaaaaaou
556   lvc250f120eaaaaaaaio   lvc250f120eaaaaaaaio
557   lvc250f120eaaaaaaaou   lvc250f120eaaaaaaaou
558   lvc250f120faaaaaaaio   lvc250f120faaaaaaaio
559   lvc250f120faaaaaaaou   lvc250f120faaaaaaaou
560   lvc250f120gaaaaaaaio   lvc250f120gaaaaaaaio
561   lvc250f120gaaaaaaaou   lvc250f120gaaaaaaaou
562   lvc250f120haaaaaaaio   lvc250f120haaaaaaaio
563   lvc250f120haaaaaaaou   lvc250f120haaaaaaaou
564   lvc250f160afaaaaaaod   lvc250f160afaaaaaaod
565   lvc250s040afaaaaaaod   lvc250s040afaaaaaaod
566   lvc250s040aaaaaaaaio   lvc250s040aaaaaaaaio
567   lvc250s040agaaaaaaod   lvc250s040agaaaaaaod
568   lvc250s040aaaaaaaaou   lvc250s040aaaaaaaaou
569   lvc250s040ahaaaaaaod   lvc250s040ahaaaaaaod
570   lvc250s040aiaaaaaaod   lvc250s040aiaaaaaaod
571   lvc250s040ajaaaaaaod   lvc250s040ajaaaaaaod
572   lvc250s040baaaaaaaio   lvc250s040baaaaaaaio
573   lvc250s040baaaaaaaou   lvc250s040baaaaaaaou
574   lvc250s040caaaaaaaio   lvc250s040caaaaaaaio
575   lvc250s040caaaaaaaou   lvc250s040caaaaaaaou
576   lvc250s040daaaaaaaio   lvc250s040daaaaaaaio
577   lvc250s040daaaaaaaou   lvc250s040daaaaaaaou
578   lvc250s040eaaaaaaaio   lvc250s040eaaaaaaaio
579   lvc250s040eaaaaaaaou   lvc250s040eaaaaaaaou
580   lvc250s040faaaaaaaio   lvc250s040faaaaaaaio
581   lvc250s040faaaaaaaou   lvc250s040faaaaaaaou
582   lvc250s040gaaaaaaaio   lvc250s040gaaaaaaaio
583   lvc250s040gaaaaaaaou   lvc250s040gaaaaaaaou
584   lvc250s040haaaaaaaio   lvc250s040haaaaaaaio
585   lvc250s040haaaaaaaou   lvc250s040haaaaaaaou
586   lvc250s080afaaaaaaod   lvc250s080afaaaaaaod
587   lvc250s080aaaaaaaaio   lvc250s080aaaaaaaaio
588   lvc250s080agaaaaaaod   lvc250s080agaaaaaaod
589   lvc250s080aaaaaaaaou   lvc250s080aaaaaaaaou
590   lvc250s080ahaaaaaaod   lvc250s080ahaaaaaaod
591   lvc250s080aiaaaaaaod   lvc250s080aiaaaaaaod
592   lvc250s080ajaaaaaaod   lvc250s080ajaaaaaaod
593   lvc250s080baaaaaaaio   lvc250s080baaaaaaaio
594   lvc250s080baaaaaaaou   lvc250s080baaaaaaaou
595   lvc250s080caaaaaaaio   lvc250s080caaaaaaaio
596   lvc250s080caaaaaaaou   lvc250s080caaaaaaaou
597   lvc250s080daaaaaaaio   lvc250s080daaaaaaaio
598   lvc250s080daaaaaaaou   lvc250s080daaaaaaaou
599   lvc250s080eaaaaaaaio   lvc250s080eaaaaaaaio
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[Diff pin]  inv_pin  vdiff  tdelay_typ  tdelay_min  tdelay_max
1   2   NA   NA   NA   NA
3   4   NA   NA   NA   NA
5   6   NA   NA   NA   NA
7   8   NA   NA   NA   NA
9   10   NA   NA   NA   NA
11   12   NA   NA   NA   NA
13   14   NA   NA   NA   NA
15   16   NA   NA   NA   NA
17   18   NA   NA   NA   NA
19   20   0.1   0.0s   0.0s   0.0s
21   22   NA   NA   NA   NA
23   24   0.1   0.0s   0.0s   0.0s
25   26   NA   NA   NA   NA
27   28   0.1   0.0s   0.0s   0.0s
29   30   NA   NA   NA   NA
31   32   0.1   0.0s   0.0s   0.0s
45   46   NA   NA   NA   NA
47   48   NA   NA   NA   NA
49   50   NA   NA   NA   NA
51   52   0.1   0.0s   0.0s   0.0s
53   54   NA   NA   NA   NA
55   56   0.1   0.0s   0.0s   0.0s
57   58   NA   NA   NA   NA
59   60   0.1   0.0s   0.0s   0.0s
61   62   NA   NA   NA   NA
63   64   0.1   0.0s   0.0s   0.0s
65   66   NA   NA   NA   NA
67   68   0.1   0.0s   0.0s   0.0s
69   70   NA   NA   NA   NA
71   72   0.1   0.0s   0.0s   0.0s
73   74   NA   NA   NA   NA
75   76   0.1   0.0s   0.0s   0.0s
77   78   NA   NA   NA   NA
79   80   0.1   0.0s   0.0s   0.0s
81   82   NA   NA   NA   NA
83   84   0.1   0.0s   0.0s   0.0s
85   86   NA   NA   NA   NA
87   88   0.1   0.0s   0.0s   0.0s
89   90   NA   NA   NA   NA
91   92   0.1   0.0s   0.0s   0.0s
93   94   NA   NA   NA   NA
95   96   0.1   0.0s   0.0s   0.0s
97   98   NA   NA   NA   NA
99   100   0.1   0.0s   0.0s   0.0s
101   102   NA   NA   NA   NA
103   104   0.1   0.0s   0.0s   0.0s
105   106   NA   NA   NA   NA
107   108   0.1   0.0s   0.0s   0.0s
109   110   NA   NA   NA   NA
111   112   0.1   0.0s   0.0s   0.0s
799   800   NA   NA   NA   NA
801   802   NA   NA   NA   NA
803   804   NA   NA   NA   NA
805   806   NA   NA   NA   NA
807   808   NA   NA   NA   NA
809   810   NA   NA   NA   NA
811   812   NA   NA   NA   NA
813   814   0.1   0.0s   0.0s   0.0s
815   816   NA   NA   NA   NA
817   818   0.1   0.0s   0.0s   0.0s
819   820   NA   NA   NA   NA
821   822   0.1   0.0s   0.0s   0.0s
823   824   NA   NA   NA   NA
825   826   0.1   0.0s   0.0s   0.0s
827   828   NA   NA   NA   NA
829   830   0.1   0.0s   0.0s   0.0s
831   832   NA   NA   NA   NA
833   834   0.1   0.0s   0.0s   0.0s
835   836   NA   NA   NA   NA
837   838   0.1   0.0s   0.0s   0.0s
839   840   NA   NA   NA   NA
841   842   0.1   0.0s   0.0s   0.0s
843   844   NA   NA   NA   NA
845   846   0.1   0.0s   0.0s   0.0s
847   848   NA   NA   NA   NA
849   850   0.1   0.0s   0.0s   0.0s
851   852   NA   NA   NA   NA
853   854   0.1   0.0s   0.0s   0.0s
855   856   NA   NA   NA   NA
857   858   0.1   0.0s   0.0s   0.0s
859   860   NA   NA   NA   NA
861   862   NA   NA   NA   NA
863   864   NA   NA   NA   NA
865   866   NA   NA   NA   NA
867   868   NA   NA   NA   NA
869   870   0.1   0.0s   0.0s   0.0s
871   872   NA   NA   NA   NA
873   874   0.1   0.0s   0.0s   0.0s
875   876   NA   NA   NA   NA
877   878   0.1   0.0s   0.0s   0.0s
879   880   NA   NA   NA   NA
881   882   0.1   0.0s   0.0s   0.0s
883   884   NA   NA   NA   NA
885   886   0.1   0.0s   0.0s   0.0s
887   888   NA   NA   NA   NA
889   890   0.1   0.0s   0.0s   0.0s
891   892   NA   NA   NA   NA
893   894   0.1   0.0s   0.0s   0.0s
895   896   NA   NA   NA   NA
897   898   0.1   0.0s   0.0s   0.0s
899   900   NA   NA   NA   NA
901   902   0.1   0.0s   0.0s   0.0s
903   904   NA   NA   NA   NA
905   906   0.1   0.0s   0.0s   0.0s
907   908   NA   NA   NA   NA
909   910   0.1   0.0s   0.0s   0.0s
911   912   NA   NA   NA   NA
913   914   0.1   0.0s   0.0s   0.0s
915   916   NA   NA   NA   NA
917   918   NA   NA   NA   NA
919   920   NA   NA   NA   NA
921   922   0.1   0.0s   0.0s   0.0s
923   924   NA   NA   NA   NA
925   926   0.1   0.0s   0.0s   0.0s
927   928   NA   NA   NA   NA
929   930   0.1   0.0s   0.0s   0.0s
931   932   NA   NA   NA   NA
933   934   0.1   0.0s   0.0s   0.0s
935   936   NA   NA   NA   NA
937   938   0.1   0.0s   0.0s   0.0s
939   940   NA   NA   NA   NA
941   942   0.1   0.0s   0.0s   0.0s
943   944   NA   NA   NA   NA
945   946   0.1   0.0s   0.0s   0.0s
947   948   NA   NA   NA   NA
949   950   0.1   0.0s   0.0s   0.0s
951   952   NA   NA   NA   NA
953   954   0.1   0.0s   0.0s   0.0s
955   956   NA   NA   NA   NA
957   958   0.1   0.0s   0.0s   0.0s
959   960   NA   NA   NA   NA
961   962   0.1   0.0s   0.0s   0.0s
963   964   NA   NA   NA   NA
965   966   0.1   0.0s   0.0s   0.0s
967   968   NA   NA   NA   NA
969   970   0.1   0.0s   0.0s   0.0s
971   972   NA   NA   NA   NA
973   974   0.1   0.0s   0.0s   0.0s
975   976   NA   NA   NA   NA
977   978   0.1   0.0s   0.0s   0.0s
979   980   NA   NA   NA   NA
981   982   0.1   0.0s   0.0s   0.0s
983   984   NA   NA   NA   NA
985   986   NA   NA   NA   NA
987   988   NA   NA   NA   NA
989   990   NA   NA   NA   NA
991   992   NA   NA   NA   NA
993   994   NA   NA   NA   NA
995   996   NA   NA   NA   NA
997   998   NA   NA   NA   NA
999   1000   NA   NA   NA   NA
1001   1002   NA   NA   NA   NA
1003   1004   NA   NA   NA   NA
1005   1006   NA   NA   NA   NA
1007   1008   NA   NA   NA   NA
1009   1010   NA   NA   NA   NA
1011   1012   NA   NA   NA   NA
1013   1014   NA   NA   NA   NA
1097   1098   NA   NA   NA   NA
1099   1100   NA   NA   NA   NA
1101   1102   NA   NA   NA   NA
1103   1104   0.1   0.0s   0.0s   0.0s
1105   1106   NA   NA   NA   NA
1107   1108   NA   NA   NA   NA
1109   1110   NA   NA   NA   NA
1111   1112   NA   NA   NA   NA
1113   1114   0.1   0.0s   0.0s   0.0s
1115   1116   NA   NA   NA   NA
1289   1290   NA   NA   NA   NA
1291   1292   NA   NA   NA   NA
1293   1294   NA   NA   NA   NA
1295   1296   NA   NA   NA   NA
1297   1298   NA   NA   NA   NA
1299   1300   NA   NA   NA   NA
1301   1302   NA   NA   NA   NA
1303   1304   NA   NA   NA   NA
1305   1306   NA   NA   NA   NA
1307   1308   NA   NA   NA   NA
1309   1310   NA   NA   NA   NA
1311   1312   NA   NA   NA   NA
1313   1314   NA   NA   NA   NA
1315   1316   NA   NA   NA   NA
1317   1318   NA   NA   NA   NA
1319   1320   NA   NA   NA   NA
1321   1322   NA   NA   NA   NA
1323   1324   NA   NA   NA   NA
1325   1326   NA   NA   NA   NA
1327   1328   NA   NA   NA   NA
1329   1330   NA   NA   NA   NA
1331   1332   NA   NA   NA   NA
1333   1334   NA   NA   NA   NA
1335   1336   NA   NA   NA   NA
1337   1338   NA   NA   NA   NA
1339   1340   NA   NA   NA   NA
1341   1342   NA   NA   NA   NA
1343   1344   NA   NA   NA   NA
1345   1346   NA   NA   NA   NA
1347   1348   NA   NA   NA   NA
1349   1350   NA   NA   NA   NA
1351   1352   NA   NA   NA   NA
1353   1354   NA   NA   NA   NA
1355   1356   NA   NA   NA   NA
1357   1358   NA   NA   NA   NA
1359   1360   NA   NA   NA   NA
[Series Pin Mapping]  pin_2   model_name   function_table_group
3   4   lvss
7   8   lvss
11   12   lvss
15   16   lvss
993   994   lvss
997   998   lvss
1001   1002   lvss
1005   1006   lvss
1099   1100   lvss
1105   1106   lvss
1109   1110   lvss
1115   1116   lvss
1307   1308   lvss
1311   1312   lvss
1315   1316   lvss
1319   1320   lvss
1347   1348   lvss
1351   1352   lvss
1355   1356   lvss
1359   1360   lvss
[Model]  lvss
Model_type   Series
C_comp   0  0  0
[Voltage Range]  1.8   1.75   1.85
[R Series]   100   110   90
|End [Model]
|End [Component]
| Models and submodels in the file (1157): blv250axxxafaaaaaain (Input), blv250axxxafaaaabain (Input), blv250axxxagaaaaaain (Input), blv250axxxagaaaabain (Input), blv250axxxefaaaaaain (Input), blv250axxxefaaaabain (Input), blv250axxxegaaaaaain (Input), blv250axxxegaaaabain (Input), blv250f160aaaaaaaaio (I/O), blv250f160aaaaaaaaou (Output), blv250f160eaaaaaaaio (I/O), blv250f160eaaaaaaaou (Output), blv250s160aaaaaaaaio (I/O), blv250s160aaaaaaaaou (Output), blv250s160eaaaaaaaio (I/O), blv250s160eaaaaaaaou (Output), i3c120f020aaaaaaaaio (I/O), i3c120f020eaaaaaaaio (I/O), i3c120s020aaaaaaaaio (I/O), i3c120s020eaaaaaaaio (I/O), i3c180f040aaaaaaaaio (I/O), i3c180f040eaaaaaaaio (I/O), i3c180s040aaaaaaaaio (I/O), i3c180s040eaaaaaaaio (I/O), i3c330f040aaaaaaaaio (I/O), i3c330f040eaaaaaaaio (I/O), i3c330s040aaaaaaaaio (I/O), i3c330s040eaaaaaaaio (I/O), ltd330axxxafaaaaaain (Input), ltd330axxxefaaaaaain (Input), ltd330f040aaaaaaaaio (I/O), ltd330f040aaaaaaaaou (Output), ltd330f040eaaaaaaaio (I/O), ltd330f040eaaaaaaaou (Output), ltd330f080aaaaaaaaio (I/O), ltd330f080aaaaaaaaou (Output), ltd330f080eaaaaaaaio (I/O), ltd330f080eaaaaaaaou (Output), ltd330f120aaaaaaaaio (I/O), ltd330f120aaaaaaaaou (Output), ltd330f120eaaaaaaaio (I/O), ltd330f120eaaaaaaaou (Output), ltd330f160aaaaaaaaio (I/O), ltd330f160aaaaaaaaou (Output), ltd330f160eaaaaaaaio (I/O), ltd330f160eaaaaaaaou (Output), ltd330s040aaaaaaaaio (I/O), ltd330s040aaaaaaaaou (Output), ltd330s040eaaaaaaaio (I/O), ltd330s040eaaaaaaaou (Output), ltd330s080aaaaaaaaio (I/O), ltd330s080aaaaaaaaou (Output), ltd330s080eaaaaaaaio (I/O), ltd330s080eaaaaaaaou (Output), ltd330s120aaaaaaaaio (I/O), ltd330s120aaaaaaaaou (Output), ltd330s120eaaaaaaaio (I/O), ltd330s120eaaaaaaaou (Output), ltd330s160aaaaaaaaio (I/O), ltd330s160aaaaaaaaou (Output), ltd330s160eaaaaaaaio (I/O), ltd330s160eaaaaaaaou (Output), lvc120axxxafaaaaaain (Input), lvc120axxxagaaaaaain (Input), lvc120axxxahaaaaaain (Input), lvc120axxxaiaaaaaain (Input), lvc120axxxbjaaaaaain (Input), lvc120axxxcfaaaaaain (Input), lvc120axxxcgaaaaaain (Input), lvc120axxxchaaaaaain (Input), lvc120axxxciaaaaaain (Input), lvc120axxxdjaaaaaain (Input), lvc120axxxefaaaaaain (Input), lvc120axxxegaaaaaain (Input), lvc120axxxehaaaaaain (Input), lvc120axxxeiaaaaaain (Input), lvc120axxxejaaaaaain (Input), lvc120axxxfjaaaaaain (Input), lvc120axxxgfaaaaaain (Input), lvc120axxxggaaaaaain (Input)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
